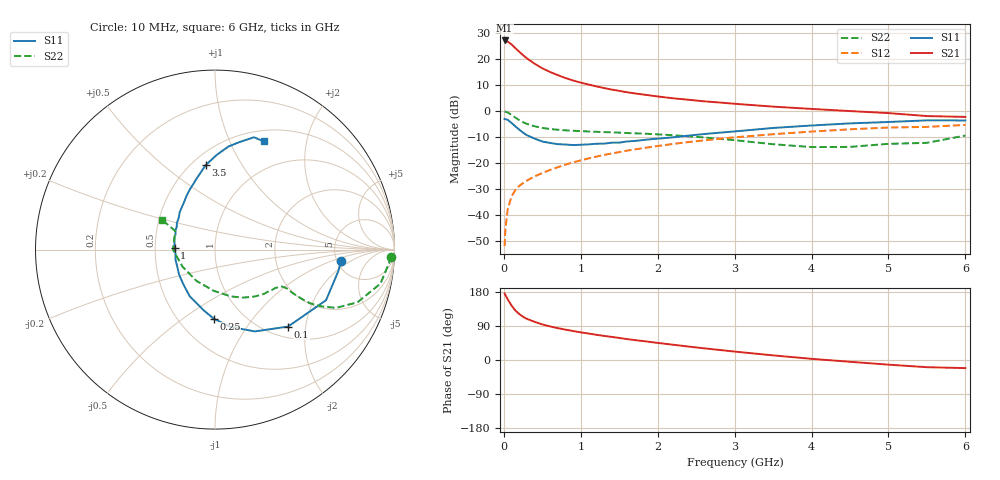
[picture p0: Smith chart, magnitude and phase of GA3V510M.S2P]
! Infineon Technologies  Discrete & RF Semiconductors
! BF775
! Si NPN RF Bipolar Junction Transistor in SOT23
! VCE = 3.5 V  IC = 10 mA
! Common Emitter S-Parameters:  May  1996
# GHz  S  MA  R  50
!  f  S11  S21  S12  S22
! GHz  MAG  ANG  MAG  ANG  MAG  ANG  MAG  ANG
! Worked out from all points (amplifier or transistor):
!   36 points, 10 MHz to 6 GHz, reference 50 ohm
!   highest |S21| = 27.2 dB at 10 MHz (marker M1)
!   |S21| within 3 dB of that: start of sweep to 151.5 MHz
!   unconditionally stable (mu >= 1): 570.3 MHz to 3.257 GHz
!   at 250 MHz: K = 0.69, MSG = 24.6 dB, |S12| = -27.7 dB
!   at 1.4 GHz: K = 1.11, MAG = 10.3 dB, |S12| = -16.3 dB
!   at 6 GHz: K = 0.95, MSG = 1.5 dB, |S12| = -5.3 dB
!   S11 on the Smith chart (normalised r, x): 10 MHz: 5.43, -1.35; 100 MHz: 1.21, -1.60; 250 MHz: 0.73, -0.66; 1 GHz: 0.63, +0.01; 3.5 GHz: 0.58, +0.71; 6 GHz: 0.63, +1.35
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0.01  0.7051 -5.1  22.94 175.8  0.0025 85.5  0.9836 -2.3
0.02  0.6975 -9.9  22.68 171.6  0.0052 88.6  0.9706 -4.8
0.05  0.6799 -24.5  21.82 160.2  0.0127 77.3  0.9413 -11.6
0.1  0.5913 -46.5  19.29 143.9  0.0227 70.1  0.8465 -20.3
0.15  0.5072 -64.0  16.32 130.6  0.0302 64.8  0.7486 -25.7
0.2  0.4398 -78.5  13.92 121.5  0.0361 62.8  0.6716 -28.1
0.25  0.3845 -91.1  11.94 114.0  0.0411 61.8  0.6106 -29.4
0.3  0.3428 -100.9  10.38 108.5  0.0458 61.9  0.5653 -29.6
0.4  0.2952 -118.7  8.183 100.7  0.0552 62.4  0.5101 -29.4
0.5  0.2596 -133.6  6.674 93.9  0.064 63.4  0.474 -28.8
0.6  0.2434 -145.4  5.684 88.7  0.0734 64.1  0.4518 -28.4
0.7  0.2308 -155.7  4.933 84.1  0.0828 64.8  0.4377 -28.6
0.8  0.2271 -165.4  4.338 80.2  0.0929 64.7  0.4261 -28.9
1  0.2247 177.9  3.533 73.0  0.1124 64.3  0.4114 -30.3
1.1  0.2281 171.5  3.25 69.9  0.1225 64.1  0.405 -31.5
1.3  0.2359 159.0  2.782 63.7  0.1429 63.0  0.3938 -33.7
1.6  0.2598 144.9  2.308 55.2  0.173 60.7  0.3778 -38.1
2.2  0.3121 124.1  1.764 40.3  0.233 55.0  0.343 -49.6
3.5  0.4733 96.3  1.219 12.2  0.3583 39.4  0.2299 -91.8
4.5  0.5798 82.5  1.001 -4.7  0.4457 26.2  0.2043 -152.1
5.5  0.6625 70.9  0.802 -19.0  0.4967 11.4  0.2446 155.0
6  0.6611 65.7  0.773 -21.4  0.5415 7.4  0.3383 150.6
